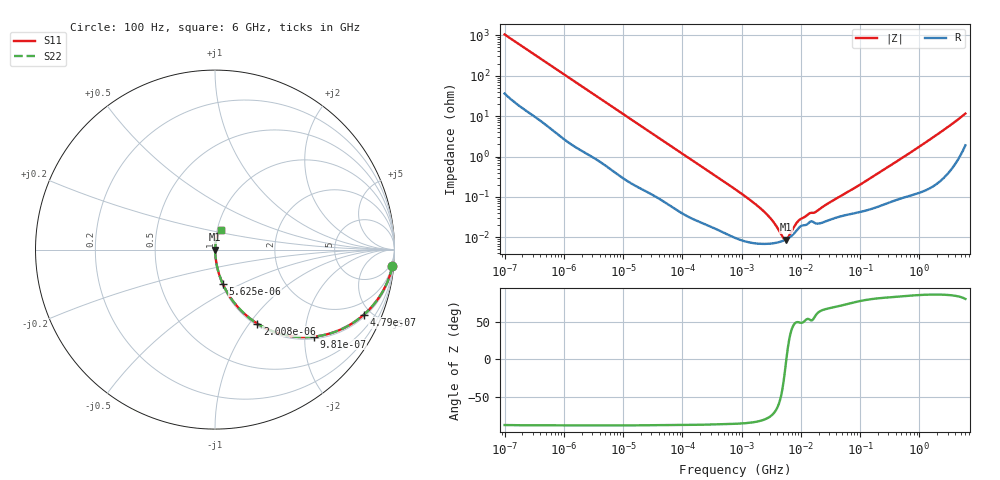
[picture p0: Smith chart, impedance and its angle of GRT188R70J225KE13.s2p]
!Murata Part Number: GRT188R70J225KE13
!These Parameters are Measured in Series Mode Connection
!Data Generated on Jun 19, 2026
!  o--ll--o
!Port1  Port2
!  o------o
!Operation Temp=25[degC], DC Bias Voltage=0[V]
!Freq. Start=100[Hz] Stop=6[GHz] 401[Steps]
# Hz S RI R 50
!Freq.(Hz) S11(Real) S11(Imag) S21(Real) S21(Imag) S12(Real) S12(Imag) S22(Real) S22(Imag)
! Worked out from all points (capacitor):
!   401 points, 100 Hz to 6 GHz, reference 50 ohm
!   read as one part in series: C = 1.51 uF near 109 Hz
!   lowest |Z| = 8.82 mohm at 5.555 MHz (marker M1)
!   series resonance near 5.704 MHz, so ESL is about 520 pH
!   S11 on the Smith chart (normalised r, x): 100 Hz: 2, -21; 479 Hz: 1.13, -4.49; 981 Hz: 1.05, -2.22; 2.008 kHz: 1.03, -1.09; 5.625 kHz: 1.01, -0.40; 6 GHz: 1.04, +0.23
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100  0.9878 -0.0938  0.0122 0.0938  0.0122 0.0938  0.9878 -0.0938
245  0.9438 -0.216  0.0562 0.216  0.0562 0.216  0.9438 -0.216
479  0.8276 -0.364  0.1724 0.364  0.1724 0.364  0.8276 -0.364
981  0.5503 -0.4852  0.4497 0.4852  0.4497 0.4852  0.5503 -0.4852
2008  0.2357 -0.4121  0.7643 0.4121  0.7643 0.4121  0.2357 -0.4121
3143  0.1167 -0.308  0.8833 0.308  0.8833 0.308  0.1167 -0.308
5625  0.0427 -0.1893  0.9573 0.1893  0.9573 0.1893  0.0427 -0.1893
13169  0.00952 -0.085  0.9905 0.085  0.9905 0.085  0.00952 -0.085
40335  0.00172 -0.0286  0.9983 0.0286  0.9983 0.0286  0.00172 -0.0286
774597  9.93e-05 -0.00156  0.9999 0.00156  0.9999 0.00156  9.93e-05 -0.00156
2372521  6.87e-05 -0.000433  0.9999 0.000433  0.9999 0.000433  6.87e-05 -0.000433
3394479  7.1e-05 -0.000237  0.9999 0.000237  0.9999 0.000237  7.1e-05 -0.000237
4856642  8.04e-05 -7.07e-05  0.9999 7.07e-05  0.9999 7.07e-05  8.04e-05 -7.07e-05
5554849  8.74e-05 -1.15e-05  0.9999 1.15e-05  0.9999 1.15e-05  8.74e-05 -1.15e-05
6353432  9.79e-05 4.76e-05  0.9999 -4.76e-05  0.9999 -4.76e-05  9.79e-05 4.76e-05
8311524  0.000141 0.000164  0.9999 -0.000164  0.9999 -0.000164  0.000141 0.000164
9506416  0.000178 0.000205  0.9998 -0.000205  0.9998 -0.000205  0.000178 0.000205
1.555665e7  0.000247 0.000317  0.9998 -0.000317  0.9998 -0.000317  0.000247 0.000317
1.86079e7  0.000218 0.000386  0.9998 -0.000386  0.9998 -0.000386  0.000218 0.000386
3.124326e8  0.00076 0.00573  0.9992 -0.00573  0.9992 -0.00573  0.00076 0.00573
1.95892e9  0.00324 0.034  0.9968 -0.034  0.9968 -0.034  0.00324 0.034
6e9  0.0307 0.1086  0.9693 -0.1086  0.9693 -0.1086  0.0307 0.1086
